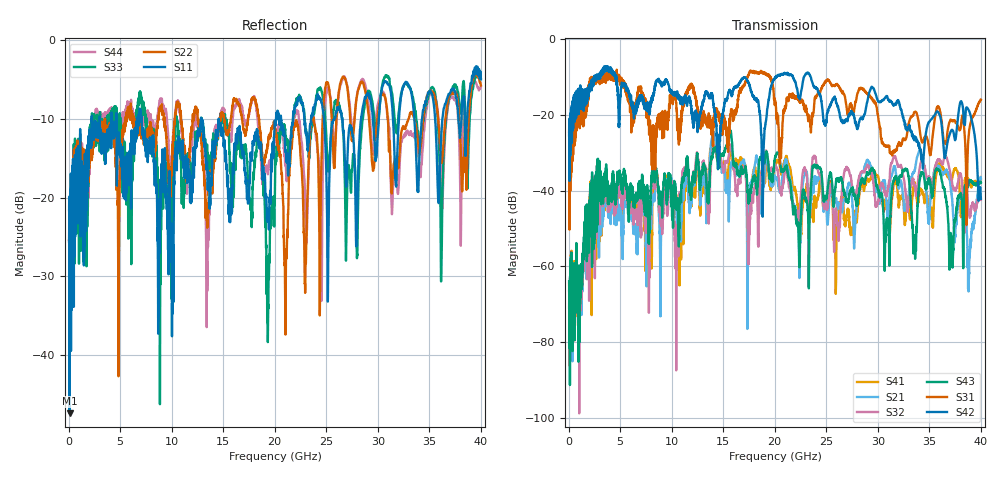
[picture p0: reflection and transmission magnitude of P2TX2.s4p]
!Agilent Technologies,N5245A,MY49151084,A.09.20.08
!Agilent N5245A: A.09.20.08
!Date: Thursday, March 01, 2012 13:17:30
!Correction: S11(Full 4 Port(1,2,3,4))
!S12(Full 4 Port(1,2,3,4))
!S13(Full 4 Port(1,2,3,4))
!S14(Full 4 Port(1,2,3,4))
!S21(Full 4 Port(1,2,3,4))
!S22(Full 4 Port(1,2,3,4))
!S23(Full 4 Port(1,2,3,4))
!S24(Full 4 Port(1,2,3,4))
!S31(Full 4 Port(1,2,3,4))
!S32(Full 4 Port(1,2,3,4))
!S33(Full 4 Port(1,2,3,4))
!S34(Full 4 Port(1,2,3,4))
!S41(Full 4 Port(1,2,3,4))
!S42(Full 4 Port(1,2,3,4))
!S43(Full 4 Port(1,2,3,4))
!S44(Full 4 Port(1,2,3,4))
!S4P File: Measurements: <S11,S12,S13,S14>,
!<S21,S22,S23,S24>,
!<S31,S32,S33,S34>,
!<S41,S42,S43,S44>:
# Hz S  dB  R 50
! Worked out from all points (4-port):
!   3996 points, 50 MHz to 40 GHz, reference 50 ohm
!   strongest paths, dB at 50 MHz, 10.04 GHz, 20.03 GHz, 30.02 GHz, 40 GHz:
!     S42: -25.4, -14.3, -10.1, -16.3, -42.2
!     S31: -24.5, -15.2, -16.2, -20.1, -16.0
!     S43: -63.9, -46.9, -31.2, -39.7, -37.9
!     S32: -70.9, -40.2, -33.1, -43.5, -42.2
!     S21: -66.6, -38.2, -36.6, -40.5, -36.7
!     S41: -64.5, -44.1, -33.4, -36.2, -37.0
!   lowest |S11| = -47.4 dB at 90 MHz (marker M1), VSWR 1.01, Z = 50.2 + j0.386 ohm
!   |S11| at or under -10 dB: start of sweep to 2.239 GHz; 7.075 GHz to 12.85 GHz (5.771 GHz wide, 57.9 % of centre); 14.56 GHz to 20.12 GHz (5.563 GHz wide, 32.1 % of centre)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
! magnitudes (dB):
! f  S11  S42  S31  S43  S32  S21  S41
! 50 MHz  -21.6  -25.4  -24.5  -63.9  -70.9  -66.6  -64.5
! 90 MHz  -47.4  -37.5  -50.3  -68.9  -75.4  -71.5  -70.5
! 2.92 GHz  -11.0  -9.3  -10.7  -33.1  -34.3  -39.2  -36.1
! 10.5 GHz  -16.5  -14.6  -18.9  -42.8  -52.0  -49.6  -45.7
! 14.04 GHz  -14.1  -17.3  -23.4  -29.7  -28.7  -24.5  -26.8
! 22.36 GHz  -7.2  -15.5  -16.3  -55.3  -48.0  -57.7  -50.6
! 40 GHz  -5.0  -42.2  -16.0  -37.9  -42.2  -36.7  -37.0
